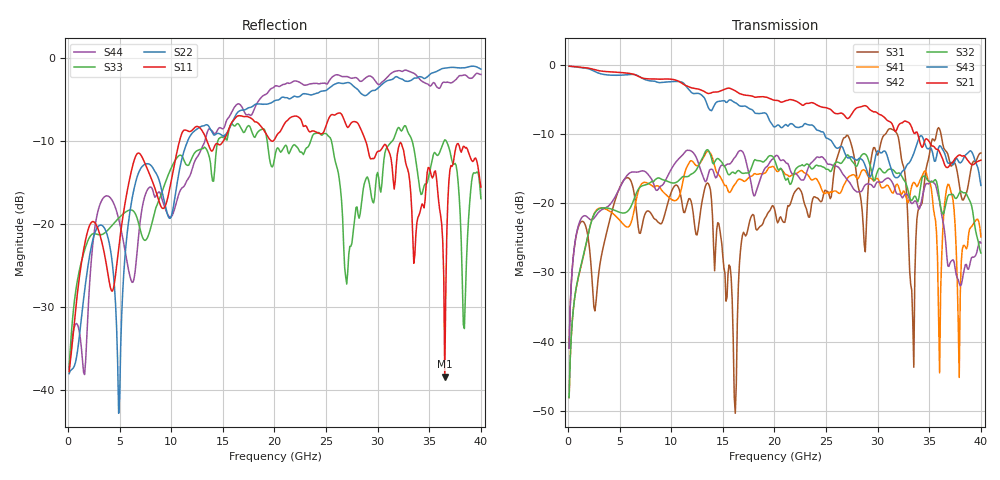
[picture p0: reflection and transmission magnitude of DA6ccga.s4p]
! ADC12DJ3200QML-SP
! 196-pin NWE package
! CCGA Ceramic Package with columns (ceramic column grid array)
! Texas Instruments 4/21/2021
! Single-ended  S-parameters
! PORT#  PORT_NAME  NET_NAME
! PORT1:  DAxN.DIEBUMP DAxN
! PORT2:  DAxN.BGA  DAxN
! PORT3:  DAxP.DIEBUMP DAxP
! PORT4:  DAxP.BGA  DAxP
! Touchstone Ver. 1.0
! Number of ports is 4
# Hz	S	MA	R	50.000000
! SCATTERING PARAMETERS  :
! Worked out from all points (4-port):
!   400 points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, 100 MHz to 40 GHz, reference 50 ohm
!   strongest paths, dB at 100 MHz, 10.1 GHz, 20.1 GHz, 30.1 GHz, 40 GHz:
!     S21: -0.1, -2.0, -5.1, -7.1, -13.7
!     S43: -0.1, -2.3, -8.9, -12.4, -17.4
!     S32: -48.1, -17.0, -14.1, -15.0, -27.2
!     S42: -41.0, -14.8, -13.1, -16.9, -25.7
!     S41: -48.1, -19.5, -15.1, -16.6, -24.8
!     S31: -40.9, -18.0, -21.5, -12.7, -12.7
!   lowest |S11| = -38.4 dB at 36.5 GHz (marker M1), VSWR 1.02, Z = 50.9 + j0.84 ohm
!   |S11| at or under -10 dB: start of sweep to 10.8 GHz; 13.46 GHz to 15.05 GHz (1.597 GHz wide, 11.2 % of centre); 28.83 GHz to end of sweep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
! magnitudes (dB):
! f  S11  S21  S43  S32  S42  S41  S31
! 100 MHz  -37.8  -0.1  -0.1  -48.1  -41.0  -48.1  -40.9
! 13.5 GHz  -10.1  -4.0  -5.8  -12.2  -16.3  -12.5  -17.0
! 16.2 GHz  -7.3  -3.7  -5.4  -15.7  -13.3  -17.2  -50.4
! 26.3 GHz  -6.6  -7.0  -11.9  -14.1  -14.9  -18.6  -12.3
! 33.5 GHz  -24.7  -9.8  -12.7  -19.1  -19.8  -16.9  -43.7
! 36.5 GHz  -38.4  -14.5  -12.8  -20.8  -24.3  -19.8  -12.2
! 40 GHz  -15.6  -13.7  -17.4  -27.2  -25.7  -24.8  -12.7
